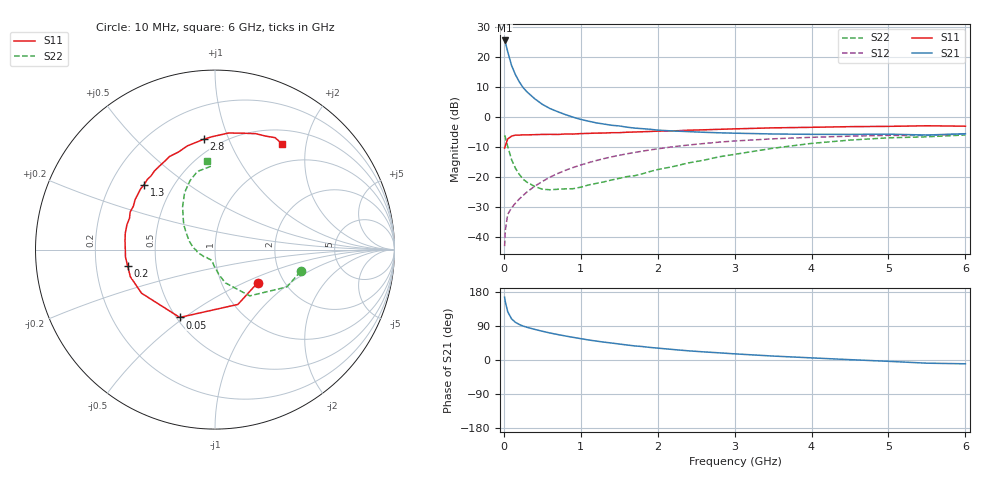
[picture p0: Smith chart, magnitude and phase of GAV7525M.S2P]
! Infineon Technologies  Discrete & RF Semiconductors
! BF775
! Si NPN RF Bipolar Junction Transistor in SOT23
! VCE = 0.75 V  IC = 25 mA
! Common Emitter S-Parameters:  May  1996
# GHz  S  MA  R  50
!  f  S11  S21  S12  S22
! GHz  MAG  ANG  MAG  ANG  MAG  ANG  MAG  ANG
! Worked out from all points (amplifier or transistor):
!   36 points, 10 MHz to 6 GHz, reference 50 ohm
!   highest |S21| = 25.4 dB at 10 MHz (marker M1)
!   |S21| within 3 dB of that: start of sweep to 42.89 MHz
!   unconditionally stable (mu >= 1): start of sweep to end of sweep
!   at 250 MHz: K = 2.52, MAG = 11.1 dB, |S12| = -26.2 dB
!   at 1.4 GHz: K = 2.37, MAG = -1.3 dB, |S12| = -13.4 dB
!   at 6 GHz: K = 1.19, MAG = -2.6 dB, |S12| = -5.7 dB
!   S11 on the Smith chart (normalised r, x): 10 MHz: 1.48, -0.60; 50 MHz: 0.52, -0.48; 200 MHz: 0.34, -0.08; 1.3 GHz: 0.34, +0.35; 2.8 GHz: 0.41, +0.82; 6 GHz: 0.70, +1.60
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0.01  0.301 -37.6  18.67 165.7  0.007 70.0  0.4923 -14.3
0.02  0.331 -67.3  17.26 153.0  0.013 63.9  0.4517 -27.4
0.05  0.426 -117.5  12.16 127.6  0.0237 51.9  0.3224 -53.1
0.1  0.4759 -149.3  7.184 108.6  0.0304 48.8  0.194 -72.7
0.15  0.4953 -162.2  5.05 99.5  0.0363 51.4  0.1395 -81.5
0.2  0.4952 -169.6  3.835 93.8  0.0427 54.2  0.1101 -86.8
0.25  0.5005 -175.2  3.07 89.6  0.0489 57.5  0.0915 -92.9
0.3  0.4996 -179.3  2.606 86.4  0.0558 60.2  0.0814 -96.5
0.4  0.5038 174.3  2.003 80.9  0.0696 62.8  0.0693 -102.0
0.5  0.5082 169.5  1.613 75.9  0.0835 64.4  0.0622 -109.9
0.6  0.51 164.1  1.371 71.3  0.0988 64.6  0.0609 -117.5
0.7  0.5074 159.9  1.215 67.2  0.1135 64.6  0.062 -124.1
0.9  0.5152 152.0  0.985 59.8  0.1429 63.0  0.0634 -135.5
1.1  0.5291 144.2  0.845 52.9  0.1719 60.9  0.0732 -147.9
1.3  0.5358 137.4  0.757 47.2  0.2009 58.2  0.0824 -160.0
1.7  0.5576 124.4  0.648 37.2  0.2545 52.1  0.1044 -178.3
2.2  0.5808 110.4  0.58 27.7  0.3167 43.8  0.1481 162.8
2.8  0.6185 95.6  0.541 18.9  0.3784 33.7  0.2157 142.7
3.5  0.6541 83.3  0.517 10.4  0.4295 22.4  0.2993 127.1
4.5  0.6847 70.6  0.509 0.9  0.4756 8.6  0.4092 109.8
5.5  0.7079 61.8  0.497 -8.4  0.4891 -3.6  0.4636 93.2
6  0.6972 57.5  0.522 -10.0  0.5185 -7.2  0.4982 95.2
